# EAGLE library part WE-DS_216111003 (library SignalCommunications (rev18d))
WE-DS D-SUB-Filter, Solder Pin Straight Characteristics Standard type filtered with 1000 pF High attenuation: max. ≥ 40 dB @ 180 MHz Choice of UNC 4/40 or through hole Rated voltage: 100 VDC Rated current @ 20 ºC: 5 A Withstand voltage: 250 VRMS Insulation resistance: min. 1000 MΩ Operating temperature: –55 ºC to +125 ºC Applications Filtering of interfaces External connection to -printer -sensor -display Details see: http://katalog.we-online.de/en/pbs/Filter_gerade Created on 2015-05-04 2015 (C) Wurth Elektronik
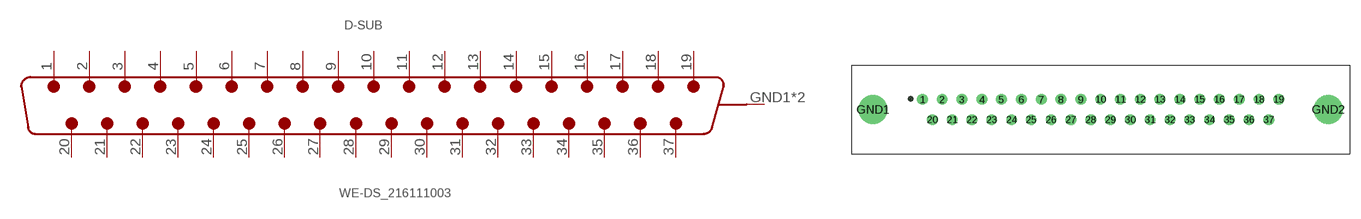
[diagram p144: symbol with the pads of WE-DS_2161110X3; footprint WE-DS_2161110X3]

Designator prefix D-SUB

## WE-DS_216111003 (WE-NUMBER: 216111003/37pins_male)  [WE-DS_2161110X3]
1  1  pas
2  2  pas
3  3  pas
4  4  pas
5  5  pas
6  6  pas
7  7  pas
8  8  pas
9  9  pas
10  10  pas
11  11  pas
12  12  pas
13  13  pas
14  14  pas
15  15  pas
16  16  pas
17  17  pas
18  18  pas
19  19  pas
20  20  pas
21  21  pas
22  22  pas
23  23  pas
24  24  pas
25  25  pas
26  26  pas
27  27  pas
28  28  pas
29  29  pas
30  30  pas
31  31  pas
32  32  pas
33  33  pas
34  34  pas
35  35  pas
36  36  pas
37  37  pas
GND1  GND  pwr
GND2  GND  pwr

## Footprint WE-DS_2161110X3 (pad centres in mm)
drill 1: 1 -24.84,1.42; 2 -22.1,1.42; 3 -19.33,1.42; 4 -16.56,1.42; 5 -13.82,1.42; 6 -11.05,1.42; 7 -8.28,1.42; 8 -5.54,1.42; 9 -2.77,1.42; 10 0,1.42; 11 2.77,1.42; 12 5.54,1.42; 13 8.28,1.42; 14 11.05,1.42; 15 13.82,1.42; 16 16.56,1.42; 17 19.33,1.42; 18 22.1,1.42; 19 24.84,1.42; 20 -23.47,-1.42; 21 -20.7,-1.42; 22 -17.96,-1.42; 23 -15.19,-1.42; 24 -12.42,-1.42; 25 -9.68,-1.42; 26 -6.91,-1.42; 27 -4.14,-1.42; 28 -1.38,-1.42; 29 1.38,-1.42; 30 4.14,-1.42; 31 6.91,-1.42; 32 9.68,-1.42; 33 12.42,-1.42; 34 15.19,-1.42; 35 17.96,-1.42; 36 20.7,-1.42; 37 23.47,-1.42
drill 3: GND1 -31.75,0; GND2 31.75,0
